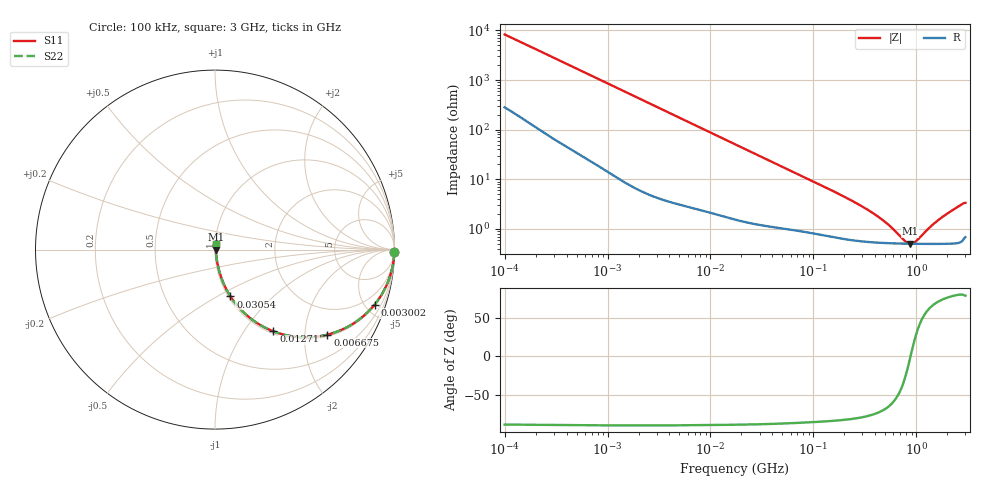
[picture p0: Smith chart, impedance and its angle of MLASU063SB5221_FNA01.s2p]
! MLASU063SB5221_FNA01  S-PARAMETER MODEL  ( Standard Model )
! Model Generated by TAIYO YUDEN Corporation (http://www.ty-top.com)
! Version 1.0
! TAIYO YUDEN Control No. 220601
! Copyright(c) 2012 TAIYO YUDEN CO.,LTD. All Rights Reserved.
! Product Description (link to TY-COMPAS)
! https://ds.yuden.co.jp/TYCOMPAS/or/detail?pn=MLASU063SB5221KFNA01&u=M
! Products Name : Multilayer Ceramic Capacitors
! Characteristics :
!  Capacitance : 220 [pF] , Rated Voltage : 50 [V] , TCC : B / X5R
!  Case Size : 0.6 x 0.3 / 0.024 x 0.012 [mm/inch] , Thickness : 0.3 / 0.012 [mm/inch]
!  (Conditions: Temperature = 25 [degC] , DC Bias Voltage = 0 [V])
! External Node Assignments :
!  1  o---| |---o  2
! GND o---------o GND
! Frequency Range : 100kHz  -  3GHz  [ 401 STEP ]
# MHZ S RI R 50
! Freq[MHz].  S11 Real  S11 Imag  S21 Real  S21 Imag  S12 Real  S12 Imag  S22 Real  S22 Imag
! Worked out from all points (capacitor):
!   401 points, 100 kHz to 3 GHz, reference 50 ohm
!   read as one part in series: C = 191 pF near 105.3 kHz
!   lowest |Z| = 501 mohm at 870.7 MHz (marker M1)
!   series resonance near 879.3 MHz, so ESL is about 170 pH
!   S11 on the Smith chart (normalised r, x): 100 kHz: open; 3.002 MHz: 1.08, -5.75; 6.675 MHz: 1.05, -2.60; 12.71 MHz: 1.04, -1.38; 30.54 MHz: 1.02, -0.58; 3 GHz: 1.01, +0.07
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0.1  0.9994 -0.012  0.000555 0.012  0.000555 0.012  0.9994 -0.012
0.562235  0.9944 -0.0654  0.00559 0.0654  0.00559 0.0654  0.9944 -0.0654
1.350433  0.9738 -0.1525  0.0262 0.1525  0.0262 0.1525  0.9738 -0.1525
3.002272  0.8887 -0.3073  0.1113 0.3073  0.1113 0.3073  0.8887 -0.3073
3.161081  0.8783 -0.3196  0.1217 0.3196  0.1217 0.3196  0.8783 -0.3196
4.534557  0.7808 -0.4053  0.2192 0.4053  0.2192 0.4053  0.7808 -0.4053
6.674626  0.6263 -0.4738  0.3737 0.4738  0.3737 0.4738  0.6263 -0.4738
9.093698  0.4793 -0.4881  0.5207 0.4881  0.5207 0.4881  0.4793 -0.4881
12.71297  0.3259 -0.4556  0.6741 0.4556  0.6741 0.4556  0.3259 -0.4556
17.7727  0.2036 -0.3876  0.7964 0.3876  0.7964 0.3876  0.2036 -0.3876
30.53531  0.0864 -0.261  0.9136 0.261  0.9136 0.261  0.0864 -0.261
53.83243  0.0356 -0.1577  0.9644 0.1577  0.9644 0.1577  0.0356 -0.1577
97.38194  0.0163 -0.0898  0.9837 0.0898  0.9837 0.0898  0.0163 -0.0898
294.964  0.00634 -0.0277  0.9937 0.0277  0.9937 0.0277  0.00634 -0.0277
412.3589  0.00556 -0.0175  0.9944 0.0175  0.9944 0.0175  0.00556 -0.0175
547.5153  0.00521 -0.0104  0.9948 0.0104  0.9948 0.0104  0.00521 -0.0104
765.4251  0.00501 -0.00294  0.995 0.00294  0.995 0.00294  0.00501 -0.00294
870.6963  0.00498 -0.000208  0.995 0.000208  0.995 0.000208  0.00498 -0.000208
990.4458  0.00497 0.00253  0.995 -0.00253  0.995 -0.00253  0.00497 0.00253
1384.641  0.00504 0.00996  0.995 -0.00996  0.995 -0.00996  0.00504 0.00996
1791.7  0.00523 0.0164  0.9948 -0.0164  0.9948 -0.0164  0.00523 0.0164
3000  0.00782 0.0323  0.9922 -0.0323  0.9922 -0.0323  0.00782 0.0323
